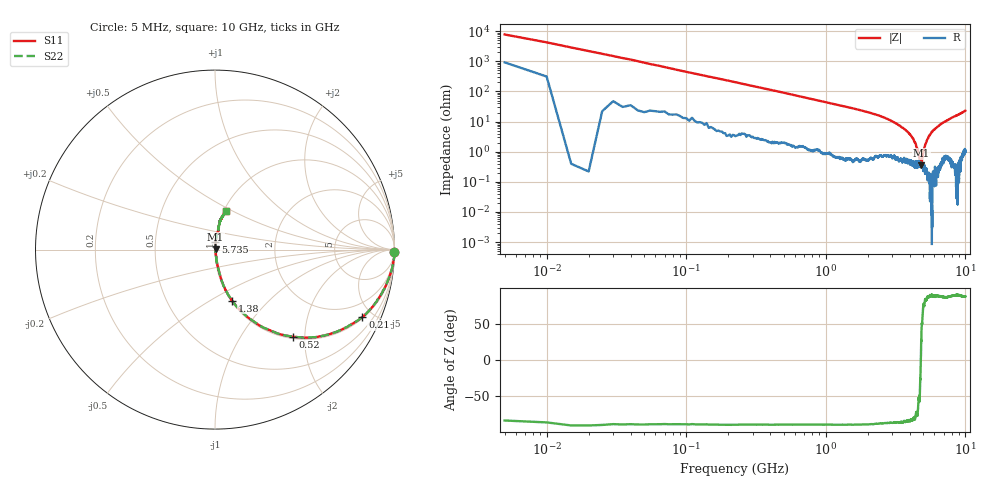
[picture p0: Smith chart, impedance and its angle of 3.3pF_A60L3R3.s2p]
! Amotech Co.,Ltd.
! http://www.amotech.co.kr/
! Part Number: A60L3R3
! These Parameters are Measured in Series Mode Connection
! Operation Temp=25[degC], DC Bias Voltage=0[V]
! Freq. Start=5[MHz] Stop=10[GHz], 2000[Steps]
! Date: Monday, July 14, 2020, 09:50:29
# GHZ S RI R 50.000000
!Freq.(Hz) S11(Real) S11(Imag) S21(Real) S21(Imag) S12(Real) S12(Imag) S22(Real) S22(Imag)
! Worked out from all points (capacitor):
!   2000 points, 5 MHz to 10 GHz, reference 50 ohm
!   read as one part in series: C = 3.54 pF near 55 MHz
!   lowest |Z| = 357 mohm at 4.825 GHz (marker M1)
!   series resonance near 4.794 GHz, so ESL is about 310 pH
!   S11 on the Smith chart (normalised r, x): 5 MHz: open; 210 MHz: 1.06, -4.35; 520 MHz: 1.04, -1.74; 1.38 GHz: 1.01, -0.63; 5.735 GHz: 1.00, +0.09; 10 GHz: 1.02, +0.47
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0.005  0.9983 -0.0127  0.00168 0.0127  0.00168 0.0127  0.9983 -0.0127
0.06  0.9792 -0.1287  0.0208 0.1287  0.0208 0.1287  0.9792 -0.1287
0.085  0.9597 -0.1808  0.0403 0.1808  0.0403 0.1808  0.9597 -0.1808
0.135  0.9124 -0.2712  0.0876 0.2712  0.0876 0.2712  0.9124 -0.2712
0.21  0.8217 -0.3756  0.1783 0.3756  0.1783 0.3756  0.8217 -0.3756
0.35  0.6268 -0.4742  0.3732 0.4742  0.3732 0.4742  0.6268 -0.4742
0.52  0.4335 -0.4849  0.5665 0.4849  0.5665 0.4849  0.4335 -0.4849
0.88  0.2102 -0.3968  0.7898 0.3968  0.7898 0.3968  0.2102 -0.3968
1.38  0.0941 -0.2839  0.9059 0.2839  0.9059 0.2839  0.0941 -0.2839
1.675  0.0657 -0.2365  0.9343 0.2365  0.9343 0.2365  0.0657 -0.2365
3.34  0.0107 -0.0742  0.9893 0.0742  0.9893 0.0742  0.0107 -0.0742
3.86  0.00618 -0.0448  0.9938 0.0448  0.9938 0.0448  0.00618 -0.0448
4.235  0.00519 -0.0259  0.9948 0.0259  0.9948 0.0259  0.00519 -0.0259
4.56  0.00391 -0.0109  0.9961 0.0109  0.9961 0.0109  0.00391 -0.0109
4.715  0.00335 -0.0037  0.9966 0.0037  0.9966 0.0037  0.00335 -0.0037
4.825  0.00315 0.00165  0.9968 -0.00165  0.9968 -0.00165  0.00315 0.00165
5.005  0.00251 0.00997  0.9975 -0.00997  0.9975 -0.00997  0.00251 0.00997
5.31  0.00238 0.0242  0.9976 -0.0242  0.9976 -0.0242  0.00238 0.0242
5.735  0.0021 0.0449  0.9979 -0.0449  0.9979 -0.0449  0.0021 0.0449
6.67  0.0107 0.0812  0.9893 -0.0812  0.9893 -0.0812  0.0107 0.0812
8.335  0.0243 0.144  0.9757 -0.144  0.9757 -0.144  0.0243 0.144
10  0.0598 0.2165  0.9402 -0.2165  0.9402 -0.2165  0.0598 0.2165
